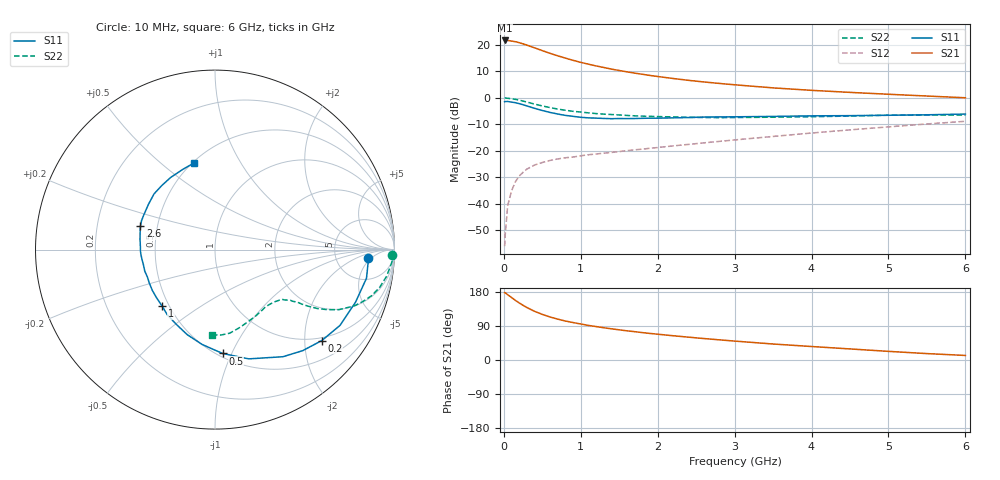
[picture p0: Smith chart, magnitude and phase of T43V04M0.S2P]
! Infineon Technologies  Discrete & RF Semiconductors
! BFR182T
! Si NPN RF Bipolar Junction Transistor in SC75
! VCE = 3 V  IC = 4 mA
! Common Emitter S-Parameters:  October  1999
# GHz  S  MA  R  50
!  f  S11  S21  S12  S22
! GHz  MAG  ANG  MAG  ANG  MAG  ANG  MAG  ANG
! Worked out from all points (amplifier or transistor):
!   36 points, 10 MHz to 6 GHz, reference 50 ohm
!   highest |S21| = 21.7 dB at 10 MHz (marker M1)
!   |S21| within 3 dB of that: start of sweep to 420.8 MHz
!   unconditionally stable (mu >= 1): 1.539 GHz to 4.078 GHz
!   at 250 MHz: K = 0.24, MSG = 24.2 dB, |S12| = -28.0 dB
!   at 1.4 GHz: K = 0.97, MSG = 15.7 dB, |S12| = -20.6 dB
!   at 6 GHz: K = 0.83, MSG = 4.4 dB, |S12| = -8.8 dB
!   S11 on the Smith chart (normalised r, x): 10 MHz: 11, -4; 200 MHz: 0.93, -2.41; 500 MHz: 0.53, -0.92; 1 GHz: 0.46, -0.36; 2.6 GHz: 0.40, +0.13; 6 GHz: 0.51, +0.65
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0.01  0.8518 -3.2  12.16 177.7  0.0016 77.4  0.9853 -1.6
0.02  0.8572 -2.9  12.08 177.2  0.0029 95.3  0.9977 -1.9
0.05  0.859 -10.7  12.15 172.2  0.0093 89.0  0.9855 -4.6
0.1  0.836 -20.5  11.86 165.0  0.0177 79.3  0.968 -8.8
0.15  0.8146 -31.2  11.52 157.3  0.0262 73.8  0.9413 -12.9
0.2  0.7817 -40.4  11.05 150.6  0.0337 71.1  0.9106 -16.3
0.25  0.7457 -49.0  10.5 144.3  0.0396 65.7  0.8725 -19.4
0.3  0.7068 -57.6  9.927 138.5  0.0456 63.4  0.8373 -22.0
0.4  0.6373 -72.8  8.831 128.4  0.0544 57.0  0.7666 -25.9
0.5  0.5803 -85.8  7.823 120.4  0.0606 54.2  0.7073 -28.2
0.6  0.5335 -97.7  6.958 113.5  0.0662 51.9  0.6591 -29.9
0.7  0.4985 -108.1  6.246 107.9  0.0707 50.5  0.6181 -31.0
0.8  0.4694 -117.2  5.651 102.9  0.0745 49.3  0.5864 -31.8
1  0.4317 -132.9  4.697 95.0  0.0812 49.8  0.5426 -32.6
1.1  0.4216 -140.9  4.34 91.2  0.0849 50.0  0.5232 -33.5
1.6  0.4076 -168.1  3.109 77.0  0.1014 52.8  0.4681 -36.4
2.2  0.4215 172.3  2.331 64.0  0.1246 56.8  0.4388 -42.2
2.6  0.4358 162.5  2.006 56.6  0.1423 58.7  0.428 -46.9
3.5  0.4487 145.5  1.55 42.2  0.188 60.3  0.4341 -58.6
4.5  0.4639 129.9  1.275 29.2  0.2503 58.9  0.4563 -72.8
5.5  0.4815 112.0  1.088 16.9  0.3234 54.8  0.4772 -86.1
6  0.4972 103.4  1.009 12.0  0.3627 51.6  0.4748 -91.8
